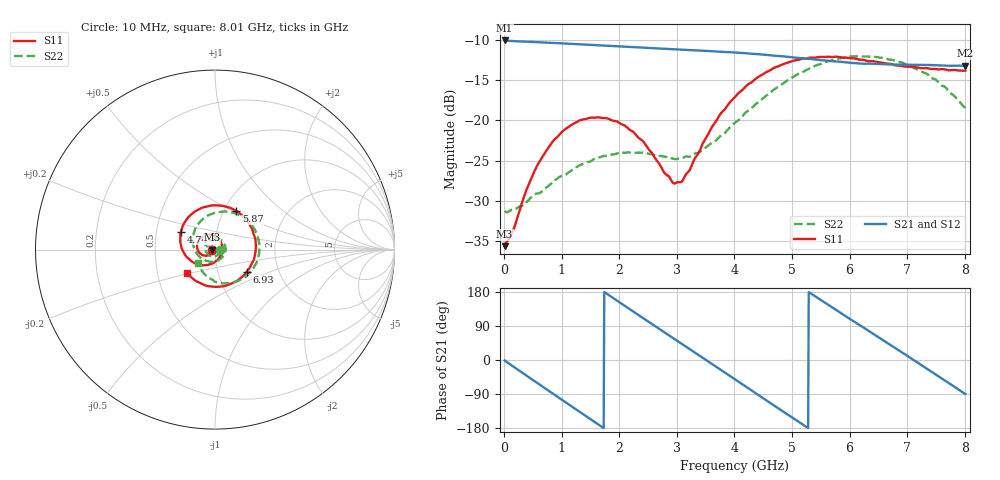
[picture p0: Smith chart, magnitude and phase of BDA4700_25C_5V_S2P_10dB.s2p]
!Agilent Technologies,E5071B,MY42404982,A.09.10
!Date: Mon Oct 20 13:31:03 2025
!Data & Calibration Information:
!Freq	S11:SOLT2(ON)	S21:SOLT2(ON)	S12:SOLT2(ON)	S22:SOLT2(ON)
# Hz S RI R 50
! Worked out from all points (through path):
!   801 points, 10 MHz to 8.01 GHz, reference 50 ohm
!   highest |S21| = -10.11 dB at 10 MHz (marker M1); lowest = -13.3 dB at 8.01 GHz (marker M2)
!   group delay of S21, straight-line fit = 280 ps
!   lowest |S11| = -35.6 dB at 10 MHz (marker M3), VSWR 1.03, Z = 48.4 - j0.125 ohm
!   |S11| at or under -10 dB: start of sweep to end of sweep
!   |S22| runs from -31.4 to -12.1 dB; largest |S21 - S12| = 0.0023
!   S11 on the Smith chart (normalised r, x): 10 MHz: 0.97, -0.00; 4.74 GHz: 0.67, +0.14; 5.87 GHz: 1.14, +0.52; 6.93 GHz: 1.38, -0.35; 8.01 GHz: 0.71, -0.20
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1e7  -0.0165 -0.00129  0.3121 -0.00691  0.312 -0.00719  0.0273 -0.00149
3.3e8  -0.024 -0.0215  0.252 -0.1761  0.2519 -0.1762  0.0217 -0.0203
7.2e8  -0.0535 -0.0343  0.0755 -0.2932  0.0758 -0.2934  -0.00367 -0.0377
1.02e9  -0.0826 -0.0221  -0.0853 -0.2869  -0.0855 -0.287  -0.0316 -0.0324
1.35e9  -0.1 0.0121  -0.2281 -0.1874  -0.2283 -0.1876  -0.0531 -0.00262
1.64e9  -0.0921 0.0489  -0.2875 -0.0486  -0.2876 -0.0487  -0.0495 0.0316
1.93e9  -0.0629 0.0763  -0.2702 0.0989  -0.2703 0.0991  -0.0227 0.0572
2.32e9  -0.00881 0.0782  -0.142 0.2442  -0.1419 0.2444  0.0268 0.057
2.68e9  0.0317 0.0444  0.0307 0.2768  0.0307 0.2766  0.0569 0.0191
2.94e9  0.0405 0.00426  0.1485 0.2317  0.1486 0.2313  0.0554 -0.016
3.08e9  0.0368 -0.0188  0.2001 0.1869  0.199 0.1877  0.0466 -0.0347
3.53e9  -0.0174 -0.0781  0.2684 -0.011  0.2686 -0.0115  -0.0122 -0.0678
4.01e9  -0.1195 -0.0716  0.1652 -0.2047  0.1653 -0.2045  -0.0886 -0.0377
4.37e9  -0.1808 -0.00369  0.0107 -0.2571  0.0105 -0.2574  -0.1226 0.0283
4.74e9  -0.1899 0.1002  -0.1448 -0.2045  -0.1444 -0.2051  -0.1096 0.1155
5.35e9  -0.0589 0.2371  -0.2372 0.0278  -0.2375 0.0272  0.0297 0.2096
5.87e9  0.1189 0.2138  -0.1209 0.1954  -0.1207 0.1952  0.1858 0.1569
6.28e9  0.211 0.1024  0.0311 0.2218  0.033 0.2211  0.2464 0.0316
6.68e9  0.2197 -0.0435  0.1636 0.1496  0.164 0.1495  0.2179 -0.096
6.93e9  0.1776 -0.1224  0.2097 0.0682  0.21 0.0675  0.1648 -0.1555
7.47e9  0.0088 -0.2075  0.178 -0.1285  0.1777 -0.1287  0.00464 -0.1805
8.01e9  -0.1543 -0.1318  -0.000131 -0.2174  0.000158 -0.2176  -0.092 -0.0745
